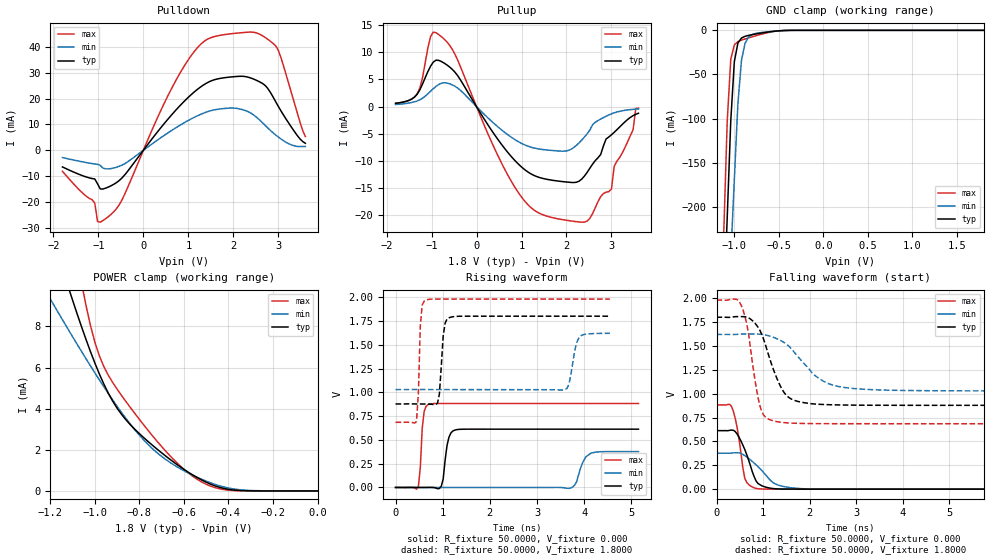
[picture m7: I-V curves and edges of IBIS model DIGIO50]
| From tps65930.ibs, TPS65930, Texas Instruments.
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|   Model DIGIO50
[Model]   DIGIO50
Model_type   I/O
Polarity   Non-Inverting
Enable   Active-Low
Vinl =   0.6900V
Vinh =   1.0500V
Vmeas =   0.9000V
Cref =  30.0000pF
Rref = 100.0000M
Vref =  0.000V
C_comp   0.4265pF   0.3732pF   0.5248pF
[Temperature Range]   25.0000   0.1250k   -40.0000
[Pullup Reference]   1.8000V   1.6200V   1.9800V
[Pulldown Reference]   0.000V   0.000V   0.000V
[POWER Clamp Reference]   1.8000V   1.6200V   1.9800V
[GND Clamp Reference]   0.000V   0.000V   0.000V
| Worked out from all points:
|   slope of the pulldown table from 0 to 0.27 V, typ, clamps not added: 43.9 ohm
|   slope of the pullup table from 0 to 0.27 V, typ, clamps not added: 76 ohm
|   GND clamp passes 1 mA (typ) near -0.55 V on its own axis
|   POWER clamp passes 1 mA (typ) near -0.59 V on its own axis
|   rising waveform, R_fixture 50.0000, V_fixture 0.000: 20-80 % time 97.7ps typ, 164ps min, 66.6ps max; typ from 0 V to 0.613 V
|   rising waveform, R_fixture 50.0000, V_fixture 1.8000: 20-80 % time 76.8ps typ, 128ps min, 51.7ps max; typ from 0.878 V to 1.8 V
|   falling waveform, R_fixture 50.0000, V_fixture 0.000: 20-80 % time 278ps typ, 458ps min, 166ps max; typ from 0.613 V to 0 V
|   falling waveform, R_fixture 50.0000, V_fixture 1.8000: 20-80 % time 414ps typ, 698ps min, 246ps max; typ from 1.8 V to 0.878 V
[Pulldown]
| voltage   I(typ)   I(min)   I(max)
-1.8V     -6.464mA   -2.835mA   -8.144mA
-1.08V    -11.12mA   -5.31mA    -20.5mA
-1.02V    -12.97mA   -5.443mA   -27.56mA
-720mV    -13.75mA   -7.086mA   -24.82mA
-480mV    -10.8mA    -5.792mA   -19.34mA
360mV     8.12mA     4.517mA    14.36mA
900mV     18.8mA     10.56mA    32.35mA
1.32V     25.06mA    14.23mA    41.71mA
1.8V      28.05mA    16.16mA    44.73mA
2.52V     26.99mA    12.68mA    45.36mA
2.94V     18.79mA    5.902mA    40.37mA
3.6V      2.682mA    1.441mA    5.304mA
[Pullup]
| voltage   I(typ)   I(min)   I(max)
-1.8V     612.8uA    402.9uA    634.7uA
-1.32V    2.285mA    1.049mA    2.357mA
-1.02V    7.473mA    2.848mA    12.94mA
-900mV    8.552mA    3.735mA    13.59mA
-480mV    6.345mA    3.755mA    9.658mA
420mV     -5.386mA   -3.317mA   -8.046mA
1.02V     -11.24mA   -6.835mA   -16.84mA
1.98V     -13.84mA   -8.168mA   -20.88mA
2.34V     -13.31mA   -6.134mA   -21.25mA
3V        -5.168mA   -1.314mA   -15.15mA
3.06V     -4.718mA   -1.134mA   -10.97mA
3.6V      -1.21mA    -414.6uA   -261.6uA
[GND_clamp]
| voltage   I(typ)   I(min)   I(max)
-1.8V     -2.195A    -1.938A    -2.466A
-1.12V    -321.9mA   -433.8mA   -233.2mA
-1.08V    -211.9mA   -345.4mA   -103.1mA
-1.04V    -102.1mA   -257mA     -32.76mA
-1V       -35.37mA   -168.6mA   -16.44mA
-960mV    -14.45mA   -82.79mA   -12.74mA
-920mV    -8.691mA   -34.07mA   -11.11mA
-880mV    -6.752mA   -14.72mA   -9.802mA
-840mV    -5.714mA   -7.575mA   -8.563mA
-680mV    -2.797mA   -2.291mA   -3.978mA
-400mV    -86.54uA   -163.3uA   -62.69uA
1.8V      130.7pA    556.4nA    175.4pA
[POWER_clamp]
| voltage   I(typ)   I(min)   I(max)
-1.8V     35.22mA    20.94mA    68.04mA
-1.22V    13.42mA    9.707mA    21.28mA
-1.2V     12.71mA    9.334mA    19.77mA
-1.1V     9.282mA    7.503mA    12.65mA
-1.06V    7.996mA    6.789mA    10.15mA
-1.04V    7.38mA     6.437mA    9.045mA
-980mV    5.697mA    5.407mA    6.58mA
-920mV    4.37mA     4.426mA    5.278mA
-760mV    2.396mA    2.25mA     2.933mA
-580mV    908.5uA    870uA      873.6uA
-420mV    120.1uA    190.9uA    65.21uA
0V        355pA      1.917nA    2.528nA
[Ramp]
| variable   typ   min   max
dV/dt_r   0.3677/96.7797p   0.1749/0.1079n   0.5294/65.9564p
dV/dt_f   0.5532/0.4099n   0.3518/0.7201n   0.7769/0.2438n
R_load = 50.0000
[Rising Waveform]
R_fixture = 50.0000
V_fixture = 0.000
V_fixture_min = 0.000
V_fixture_max = 0.000
| time   V(typ)   V(min)   V(max)
0s        6.861nV    138.8nV    15.16nV
484.8ps   114.9uV    32.72uV    11.06mV
606.1ps   164.5uV    26.84uV    798.1mV
727.3ps   784.1uV    22.72uV    877.8mV
969.7ps   13.06mV    16.61uV    882.5mV
1.131ns   526.4mV    14.1uV     882.3mV
1.252ns   602.3mV    12.29uV    882.3mV
3.677ns   612.8mV    -9.008mV   882.3mV
4.141ns   612.8mV    359.7mV    882.3mV
5.152ns   612.8mV    376.8mV    882.3mV
[Rising Waveform]
R_fixture = 50.0000
V_fixture = 1.8000
V_fixture_min = 1.6200
V_fixture_max = 1.9800
| time   V(typ)   V(min)   V(max)
0s        877.8mV    1.029V     685.2mV
444.4ps   877.8mV    1.029V     693.3mV
525.3ps   877.4mV    1.029V     1.701V
646.5ps   876.5mV    1.029V     1.97V
888.9ps   884.7mV    1.029V     1.98V
1.01ns    1.591V     1.029V     1.98V
1.131ns   1.783V     1.029V     1.98V
3.596ns   1.8V       1.028V     1.98V
3.919ns   1.8V       1.589V     1.98V
4.546ns   1.8V       1.62V      1.98V
[Falling Waveform]
R_fixture = 50.0000
V_fixture = 0.000
V_fixture_min = 0.000
V_fixture_max = 0.000
| time   V(typ)   V(min)   V(max)
0s        612.8mV    376.8mV    882.3mV
323.2ps   618.3mV    377.6mV    865.2mV
444.4ps   576.3mV    381.3mV    639.5mV
606.1ps   415.5mV    351.9mV    114.3mV
686.9ps   307.8mV    322.5mV    50.07mV
848.5ps   86.71mV    255.6mV    8.383mV
969.7ps   36.04mV    196.7mV    2.108mV
1.252ns   4.739mV    57.1mV     838.6uV
1.818ns   639uV      5.586mV    134.9uV
10ns      135.8nV    373.4nV    132.3nV
[Falling Waveform]
R_fixture = 50.0000
V_fixture = 1.8000
V_fixture_min = 1.6200
V_fixture_max = 1.9800
| time   V(typ)   V(min)   V(max)
0s        1.8V       1.62V      1.98V
525.3ps   1.807V     1.623V     1.93V
646.5ps   1.801V     1.624V     1.736V
929.3ps   1.666V     1.622V     877.2mV
1.252ns   1.213V     1.584V     711.1mV
1.455ns   1.009V     1.534V     696.7mV
1.657ns   932.7mV    1.441V     690.8mV
2.182ns   889.3mV    1.165V     686mV
2.788ns   880.7mV    1.062V     685.3mV
10ns      877.8mV    1.029V     685.2mV
